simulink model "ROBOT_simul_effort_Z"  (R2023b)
settings: Solver=VariableStepAuto  StartTime=0.0  StopTime=5  RelTol=1e-3
undefined symbols (not defined in the file): deg, kg, m, manette1_Defaut_sldprt, manette2_Defaut_sldprt, mm, N, rad, s, STL, X, Y, Z
libraries: sm_lib x463, fl_lib x45, nesl_utility x27, simulink x2
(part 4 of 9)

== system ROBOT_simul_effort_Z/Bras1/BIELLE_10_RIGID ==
  AXE_BIELLE_1_RIGID : Subsystem
  AXE_BIELLE_2_RIGID : Subsystem
  BIELLE_PARALLELOGRAMME_1_RIGID : Subsystem
  ReferenceFrame : sm_lib/Frames and Transforms/Reference Frame
  Transform : sm_lib/Frames and Transforms/Rigid Transform  TranslationMethod=Cartesian  TranslationStandardOffset=0  TranslationStandardOffsetUnits=mm  TranslationStandardAxis=+Z  TranslationCartesianOffset=[-181.1287710013672 12.999999999999993 -105.75000000000001]  TranslationCartesianOffsetUnits=mm  TranslationROffset=0  TranslationROffsetUnits=m  TranslationZOffset=0  TranslationZOffsetUnits=m  TranslationThetaOffset=0  TranslationThetaOffsetUnits=deg  RotationMethod=ArbitraryAxis  RotationAngleUnits=rad  RotationStandardAxis=+Z  RotationAngle=2.0943951023931957  RotationArbitraryAxis=[0.57735026918962573 -0.57735026918962573 0.57735026918962562]  FollAlignAxisA=+X  BaseAlignAxisA=+Y  FollAlignAxisB=+Y  BaseAlignAxisB=+Z  RotationSequenceAxes=FollowerAxes  RotationSequence=XYX  RotationSequenceAngles=[0 0 0]  RotationSequenceAnglesUnits=deg  RotationMatrix=[1 0 0; 0 1 0; 0 0 1]  Quaternion=[1 0 0 0]
  Transform1 : sm_lib/Frames and Transforms/Rigid Transform  TranslationMethod=Cartesian  TranslationStandardOffset=0  TranslationStandardOffsetUnits=mm  TranslationStandardAxis=+Z  TranslationCartesianOffset=[-181.12877100136717 13.000000000000004 -3.249999999999996]  TranslationCartesianOffsetUnits=mm  TranslationROffset=0  TranslationROffsetUnits=m  TranslationZOffset=0  TranslationZOffsetUnits=m  TranslationThetaOffset=0  TranslationThetaOffsetUnits=deg  RotationMethod=ArbitraryAxis  RotationAngleUnits=rad  RotationStandardAxis=+Z  RotationAngle=2.0943951023931953  RotationArbitraryAxis=[0.57735026918962584 -0.57735026918962584 0.57735026918962584]  FollAlignAxisA=+X  BaseAlignAxisA=+Y  FollAlignAxisB=+Y  BaseAlignAxisB=+Z  RotationSequenceAxes=FollowerAxes  RotationSequence=XYX  RotationSequenceAngles=[0 0 0]  RotationSequenceAnglesUnits=deg  RotationMatrix=[1 0 0; 0 1 0; 0 0 1]  Quaternion=[1 0 0 0]
  Transform2 : sm_lib/Frames and Transforms/Rigid Transform  TranslationMethod=Cartesian  TranslationStandardOffset=0  TranslationStandardOffsetUnits=mm  TranslationStandardAxis=+Z  TranslationCartesianOffset=[-178.12877100136717 5.0000000000000115 -54.500000000000007]  TranslationCartesianOffsetUnits=mm  TranslationROffset=0  TranslationROffsetUnits=m  TranslationZOffset=0  TranslationZOffsetUnits=m  TranslationThetaOffset=0  TranslationThetaOffsetUnits=deg  RotationMethod=ArbitraryAxis  RotationAngleUnits=rad  RotationStandardAxis=+Z  RotationAngle=3.1415926535897931  RotationArbitraryAxis=[-0.70710678118654746 0.70710678118654768 0]  FollAlignAxisA=+X  BaseAlignAxisA=+Y  FollAlignAxisB=+Y  BaseAlignAxisB=+Z  RotationSequenceAxes=FollowerAxes  RotationSequence=XYX  RotationSequenceAngles=[0 0 0]  RotationSequenceAnglesUnits=deg  RotationMatrix=[1 0 0; 0 1 0; 0 0 1]  Quaternion=[1 0 0 0]
  Transform3 : sm_lib/Frames and Transforms/Rigid Transform  TranslationMethod=Cartesian  TranslationStandardOffset=0  TranslationStandardOffsetUnits=mm  TranslationStandardAxis=+Z  TranslationCartesianOffset=[-181.1287710013672 4.999999999999984 -105.75000000000001]  TranslationCartesianOffsetUnits=mm  TranslationROffset=0  TranslationROffsetUnits=m  TranslationZOffset=0  TranslationZOffsetUnits=m  TranslationThetaOffset=0  TranslationThetaOffsetUnits=deg  RotationMethod=ArbitraryAxis  RotationAngleUnits=rad  RotationStandardAxis=+Z  RotationAngle=1.7602050674842988  RotationArbitraryAxis=[-0.82650316451596495 -0.3980530863120495 -0.3980530863120495]  FollAlignAxisA=+X  BaseAlignAxisA=+Y  FollAlignAxisB=+Y  BaseAlignAxisB=+Z  RotationSequenceAxes=FollowerAxes  RotationSequence=XYX  RotationSequenceAngles=[0 0 0]  RotationSequenceAnglesUnits=deg  RotationMatrix=[1 0 0; 0 1 0; 0 0 1]  Quaternion=[1 0 0 0]
  Transform4 : sm_lib/Frames and Transforms/Rigid Transform  TranslationMethod=Cartesian  TranslationStandardOffset=0  TranslationStandardOffsetUnits=mm  TranslationStandardAxis=+Z  TranslationCartesianOffset=[-181.12877100136717 5.0000000000000115 -3.249999999999996]  TranslationCartesianOffsetUnits=mm  TranslationROffset=0  TranslationROffsetUnits=m  TranslationZOffset=0  TranslationZOffsetUnits=m  TranslationThetaOffset=0  TranslationThetaOffsetUnits=deg  RotationMethod=ArbitraryAxis  RotationAngleUnits=rad  RotationStandardAxis=+Z  RotationAngle=1.7602050674842997  RotationArbitraryAxis=[-0.82650316451596506 -0.39805308631204933 -0.39805308631204933]  FollAlignAxisA=+X  BaseAlignAxisA=+Y  FollAlignAxisB=+Y  BaseAlignAxisB=+Z  RotationSequenceAxes=FollowerAxes  RotationSequence=XYX  RotationSequenceAngles=[0 0 0]  RotationSequenceAnglesUnits=deg  RotationMatrix=[1 0 0; 0 1 0; 0 0 1]  Quaternion=[1 0 0 0]
  F1 : PMIOPort  Side=Right
  F : PMIOPort  Port=2  Side=Left
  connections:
  Transform/LConn1 -- ReferenceFrame/RConn1 -- Transform3/LConn1 -- Transform4/LConn1 -- Transform2/LConn1 -- Transform1/LConn1
  Transform/RConn1 -- F/RConn1
  Transform1/RConn1 -- F1/RConn1
  BIELLE_PARALLELOGRAMME_1_RIGID/LConn1 -- Transform2/RConn1
  AXE_BIELLE_1_RIGID/LConn1 -- Transform3/RConn1
  AXE_BIELLE_2_RIGID/LConn1 -- Transform4/RConn1

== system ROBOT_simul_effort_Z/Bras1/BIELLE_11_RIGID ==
  AXE_BIELLE_1_RIGID : Subsystem
  AXE_BIELLE_2_RIGID : Subsystem
  BIELLE_PARALLELOGRAMME_1_RIGID : Subsystem
  ReferenceFrame : sm_lib/Frames and Transforms/Reference Frame
  Transform : sm_lib/Frames and Transforms/Rigid Transform  TranslationMethod=Cartesian  TranslationStandardOffset=0  TranslationStandardOffsetUnits=mm  TranslationStandardAxis=+Z  TranslationCartesianOffset=[-181.12877100136717 13.000000000000018 -105.75000000000001]  TranslationCartesianOffsetUnits=mm  TranslationROffset=0  TranslationROffsetUnits=m  TranslationZOffset=0  TranslationZOffsetUnits=m  TranslationThetaOffset=0  TranslationThetaOffsetUnits=deg  RotationMethod=ArbitraryAxis  RotationAngleUnits=rad  RotationStandardAxis=+Z  RotationAngle=2.0943951023931962  RotationArbitraryAxis=[0.57735026918962595 -0.57735026918962562 0.57735026918962562]  FollAlignAxisA=+X  BaseAlignAxisA=+Y  FollAlignAxisB=+Y  BaseAlignAxisB=+Z  RotationSequenceAxes=FollowerAxes  RotationSequence=XYX  RotationSequenceAngles=[0 0 0]  RotationSequenceAnglesUnits=deg  RotationMatrix=[1 0 0; 0 1 0; 0 0 1]  Quaternion=[1 0 0 0]
  Transform1 : sm_lib/Frames and Transforms/Rigid Transform  TranslationMethod=Cartesian  TranslationStandardOffset=0  TranslationStandardOffsetUnits=mm  TranslationStandardAxis=+Z  TranslationCartesianOffset=[-181.12877100136714 13.000000000000014 -3.2499999999999889]  TranslationCartesianOffsetUnits=mm  TranslationROffset=0  TranslationROffsetUnits=m  TranslationZOffset=0  TranslationZOffsetUnits=m  TranslationThetaOffset=0  TranslationThetaOffsetUnits=deg  RotationMethod=ArbitraryAxis  RotationAngleUnits=rad  RotationStandardAxis=+Z  RotationAngle=2.0943951023931957  RotationArbitraryAxis=[0.57735026918962573 -0.57735026918962562 0.57735026918962595]  FollAlignAxisA=+X  BaseAlignAxisA=+Y  FollAlignAxisB=+Y  BaseAlignAxisB=+Z  RotationSequenceAxes=FollowerAxes  RotationSequence=XYX  RotationSequenceAngles=[0 0 0]  RotationSequenceAnglesUnits=deg  RotationMatrix=[1 0 0; 0 1 0; 0 0 1]  Quaternion=[1 0 0 0]
  Transform2 : sm_lib/Frames and Transforms/Rigid Transform  TranslationMethod=Cartesian  TranslationStandardOffset=0  TranslationStandardOffsetUnits=mm  TranslationStandardAxis=+Z  TranslationCartesianOffset=[-178.12877100136714 5.0000000000000044 -54.500000000000007]  TranslationCartesianOffsetUnits=mm  TranslationROffset=0  TranslationROffsetUnits=m  TranslationZOffset=0  TranslationZOffsetUnits=m  TranslationThetaOffset=0  TranslationThetaOffsetUnits=deg  RotationMethod=ArbitraryAxis  RotationAngleUnits=rad  RotationStandardAxis=+Z  RotationAngle=3.1415926535897931  RotationArbitraryAxis=[-0.70710678118654746 0.70710678118654757 0]  FollAlignAxisA=+X  BaseAlignAxisA=+Y  FollAlignAxisB=+Y  BaseAlignAxisB=+Z  RotationSequenceAxes=FollowerAxes  RotationSequence=XYX  RotationSequenceAngles=[0 0 0]  RotationSequenceAnglesUnits=deg  RotationMatrix=[1 0 0; 0 1 0; 0 0 1]  Quaternion=[1 0 0 0]
  Transform3 : sm_lib/Frames and Transforms/Rigid Transform  TranslationMethod=Cartesian  TranslationStandardOffset=0  TranslationStandardOffsetUnits=mm  TranslationStandardAxis=+Z  TranslationCartesianOffset=[-181.12877100136717 5.0000000000000044 -105.75000000000001]  TranslationCartesianOffsetUnits=mm  TranslationROffset=0  TranslationROffsetUnits=m  TranslationZOffset=0  TranslationZOffsetUnits=m  TranslationThetaOffset=0  TranslationThetaOffsetUnits=deg  RotationMethod=ArbitraryAxis  RotationAngleUnits=rad  RotationStandardAxis=+Z  RotationAngle=1.7602050674842991  RotationArbitraryAxis=[-0.82650316451596495 -0.3980530863120495 -0.39805308631204944]  FollAlignAxisA=+X  BaseAlignAxisA=+Y  FollAlignAxisB=+Y  BaseAlignAxisB=+Z  RotationSequenceAxes=FollowerAxes  RotationSequence=XYX  RotationSequenceAngles=[0 0 0]  RotationSequenceAnglesUnits=deg  RotationMatrix=[1 0 0; 0 1 0; 0 0 1]  Quaternion=[1 0 0 0]
  Transform4 : sm_lib/Frames and Transforms/Rigid Transform  TranslationMethod=Cartesian  TranslationStandardOffset=0  TranslationStandardOffsetUnits=mm  TranslationStandardAxis=+Z  TranslationCartesianOffset=[-181.12877100136714 5.0000000000000044 -3.2499999999999889]  TranslationCartesianOffsetUnits=mm  TranslationROffset=0  TranslationROffsetUnits=m  TranslationZOffset=0  TranslationZOffsetUnits=m  TranslationThetaOffset=0  TranslationThetaOffsetUnits=deg  RotationMethod=ArbitraryAxis  RotationAngleUnits=rad  RotationStandardAxis=+Z  RotationAngle=1.7602050674842995  RotationArbitraryAxis=[-0.82650316451596506 -0.39805308631204939 -0.39805308631204933]  FollAlignAxisA=+X  BaseAlignAxisA=+Y  FollAlignAxisB=+Y  BaseAlignAxisB=+Z  RotationSequenceAxes=FollowerAxes  RotationSequence=XYX  RotationSequenceAngles=[0 0 0]  RotationSequenceAnglesUnits=deg  RotationMatrix=[1 0 0; 0 1 0; 0 0 1]  Quaternion=[1 0 0 0]
  F1 : PMIOPort  Side=Right
  F : PMIOPort  Port=2  Side=Left
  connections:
  Transform/LConn1 -- ReferenceFrame/RConn1 -- Transform3/LConn1 -- Transform4/LConn1 -- Transform2/LConn1 -- Transform1/LConn1
  Transform/RConn1 -- F/RConn1
  Transform1/RConn1 -- F1/RConn1
  BIELLE_PARALLELOGRAMME_1_RIGID/LConn1 -- Transform2/RConn1
  AXE_BIELLE_1_RIGID/LConn1 -- Transform3/RConn1
  AXE_BIELLE_2_RIGID/LConn1 -- Transform4/RConn1

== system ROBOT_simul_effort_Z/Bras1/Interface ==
  Angular Velocity Source : fl_lib/Mechanical/Mechanical Sources/Ideal Angular Velocity Source
  Torque Sensor : fl_lib/Mechanical/Mechanical Sensors/Ideal Torque Sensor
  C : PMIOPort  Side=Left
  T : PMIOPort  Port=2  Side=Right
  w : PMIOPort  Port=3  Side=Right
  R : PMIOPort  Port=4  Side=Left
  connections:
  R/RConn1 -- Angular Velocity Source/LConn1
  Torque Sensor/LConn1 -- Angular Velocity Source/RConn2
  Torque Sensor/RConn2 -- T/RConn1
  C/RConn1 -- Torque Sensor/RConn1
  Angular Velocity Source/RConn1 -- w/RConn1

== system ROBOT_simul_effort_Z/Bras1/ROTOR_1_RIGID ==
  CODEUR_1_RIGID : Subsystem
  ROTOR_1_RIGID : Subsystem
  ReferenceFrame : sm_lib/Frames and Transforms/Reference Frame
  Transform : sm_lib/Frames and Transforms/Rigid Transform  TranslationMethod=Cartesian  TranslationStandardOffset=0  TranslationStandardOffsetUnits=mm  TranslationStandardAxis=+Z  TranslationCartesianOffset=[29.900000000000013 -3.5527136788005009e-15 2.2204460492503131e-14]  TranslationCartesianOffsetUnits=mm  TranslationROffset=0  TranslationROffsetUnits=m  TranslationZOffset=0  TranslationZOffsetUnits=m  TranslationThetaOffset=0  TranslationThetaOffsetUnits=deg  RotationMethod=ArbitraryAxis  RotationAngleUnits=rad  RotationStandardAxis=+Z  RotationAngle=2.0943951023931953  RotationArbitraryAxis=[0.57735026918962595 0.57735026918962562 0.57735026918962562]  FollAlignAxisA=+X  BaseAlignAxisA=+Y  FollAlignAxisB=+Y  BaseAlignAxisB=+Z  RotationSequenceAxes=FollowerAxes  RotationSequence=XYX  RotationSequenceAngles=[0 0 0]  RotationSequenceAnglesUnits=deg  RotationMatrix=[1 0 0; 0 1 0; 0 0 1]  Quaternion=[1 0 0 0]
  Transform1 : sm_lib/Frames and Transforms/Rigid Transform  TranslationMethod=Cartesian  TranslationStandardOffset=0  TranslationStandardOffsetUnits=mm  TranslationStandardAxis=+Z  TranslationCartesianOffset=[30.899999999999981 0 0]  TranslationCartesianOffsetUnits=mm  TranslationROffset=0  TranslationROffsetUnits=m  TranslationZOffset=0  TranslationZOffsetUnits=m  TranslationThetaOffset=0  TranslationThetaOffsetUnits=deg  RotationMethod=ArbitraryAxis  RotationAngleUnits=rad  RotationStandardAxis=+Z  RotationAngle=1.9381695666920586  RotationArbitraryAxis=[0.51405666735189148 -0.51405666735189148 0.68665237602598705]  FollAlignAxisA=+X  BaseAlignAxisA=+Y  FollAlignAxisB=+Y  BaseAlignAxisB=+Z  RotationSequenceAxes=FollowerAxes  RotationSequence=XYX  RotationSequenceAngles=[0 0 0]  RotationSequenceAnglesUnits=deg  RotationMatrix=[1 0 0; 0 1 0; 0 0 1]  Quaternion=[1 0 0 0]
  Transform2 : sm_lib/Frames and Transforms/Rigid Transform  TranslationMethod=Cartesian  TranslationStandardOffset=0  TranslationStandardOffsetUnits=mm  TranslationStandardAxis=+Z  TranslationCartesianOffset=[-36.399999999999999 0 0]  TranslationCartesianOffsetUnits=mm  TranslationROffset=0  TranslationROffsetUnits=m  TranslationZOffset=0  TranslationZOffsetUnits=m  TranslationThetaOffset=0  TranslationThetaOffsetUnits=deg  RotationMethod=ArbitraryAxis  RotationAngleUnits=rad  RotationStandardAxis=+Z  RotationAngle=1.624664356272121  RotationArbitraryAxis=[-0.22603347840136145 0.22603347840136123 0.94753244444903439]  FollAlignAxisA=+X  BaseAlignAxisA=+Y  FollAlignAxisB=+Y  BaseAlignAxisB=+Z  RotationSequenceAxes=FollowerAxes  RotationSequence=XYX  RotationSequenceAngles=[0 0 0]  RotationSequenceAnglesUnits=deg  RotationMatrix=[1 0 0; 0 1 0; 0 0 1]  Quaternion=[1 0 0 0]
  F : PMIOPort  Side=Left
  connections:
  Transform/LConn1 -- ReferenceFrame/RConn1 -- Transform1/LConn1 -- Transform2/LConn1
  Transform/RConn1 -- F/RConn1
  ROTOR_1_RIGID/LConn1 -- Transform1/RConn1
  CODEUR_1_RIGID/LConn1 -- Transform2/RConn1

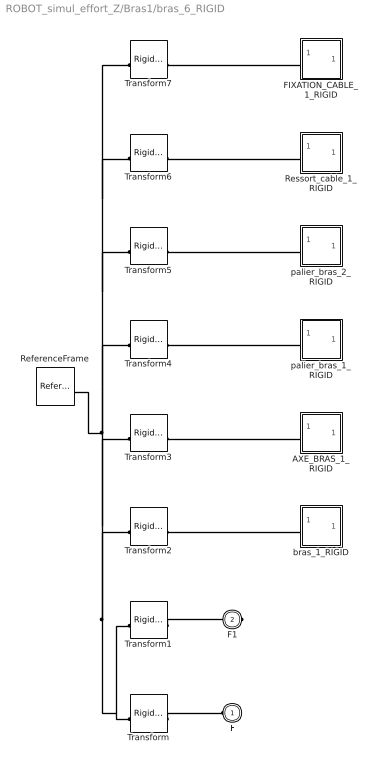
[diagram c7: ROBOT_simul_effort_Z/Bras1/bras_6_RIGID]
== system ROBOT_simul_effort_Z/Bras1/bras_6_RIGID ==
  AXE_BRAS_1_RIGID : Subsystem
  FIXATION_CABLE_1_RIGID : Subsystem
  ReferenceFrame : sm_lib/Frames and Transforms/Reference Frame
  Ressort_cable_1_RIGID : Subsystem
  Transform : sm_lib/Frames and Transforms/Rigid Transform  TranslationMethod=Cartesian  TranslationStandardOffset=0  TranslationStandardOffsetUnits=mm  TranslationStandardAxis=+Z  TranslationCartesianOffset=[-97.415569487383038 39.82561820207529 -20.980989744699272]  TranslationCartesianOffsetUnits=mm  TranslationROffset=0  TranslationROffsetUnits=m  TranslationZOffset=0  TranslationZOffsetUnits=m  TranslationThetaOffset=0  TranslationThetaOffsetUnits=deg  RotationMethod=ArbitraryAxis  RotationAngleUnits=rad  RotationStandardAxis=+Z  RotationAngle=2.0943951023931957  RotationArbitraryAxis=[-0.57735026918962551 -0.57735026918962595 0.57735026918962573]  FollAlignAxisA=+X  BaseAlignAxisA=+Y  FollAlignAxisB=+Y  BaseAlignAxisB=+Z  RotationSequenceAxes=FollowerAxes  RotationSequence=XYX  RotationSequenceAngles=[0 0 0]  RotationSequenceAnglesUnits=deg  RotationMatrix=[1 0 0; 0 1 0; 0 0 1]  Quaternion=[1 0 0 0]
  Transform1 : sm_lib/Frames and Transforms/Rigid Transform  TranslationMethod=Cartesian  TranslationStandardOffset=0  TranslationStandardOffsetUnits=mm  TranslationStandardAxis=+Z  TranslationCartesianOffset=[-176.59192436800635 99.825618202078147 -20.980989744703663]  TranslationCartesianOffsetUnits=mm  TranslationROffset=0  TranslationROffsetUnits=m  TranslationZOffset=0  TranslationZOffsetUnits=m  TranslationThetaOffset=0  TranslationThetaOffsetUnits=deg  RotationMethod=ArbitraryAxis  RotationAngleUnits=rad  RotationStandardAxis=+Z  RotationAngle=2.0943951023931953  RotationArbitraryAxis=[0.57735026918962584 0.57735026918962584 0.57735026918962584]  FollAlignAxisA=+X  BaseAlignAxisA=+Y  FollAlignAxisB=+Y  BaseAlignAxisB=+Z  RotationSequenceAxes=FollowerAxes  RotationSequence=XYX  RotationSequenceAngles=[0 0 0]  RotationSequenceAnglesUnits=deg  RotationMatrix=[1 0 0; 0 1 0; 0 0 1]  Quaternion=[1 0 0 0]
  Transform2 : sm_lib/Frames and Transforms/Rigid Transform  TranslationMethod=Cartesian  TranslationStandardOffset=0  TranslationStandardOffsetUnits=mm  TranslationStandardAxis=+Z  TranslationCartesianOffset=[-166.59192436800635 39.825618202078147 -20.98098974470366]  TranslationCartesianOffsetUnits=mm  TranslationROffset=0  TranslationROffsetUnits=m  TranslationZOffset=0  TranslationZOffsetUnits=m  TranslationThetaOffset=0  TranslationThetaOffsetUnits=deg  RotationMethod=ArbitraryAxis  RotationAngleUnits=rad  RotationStandardAxis=+Z  RotationAngle=1.5707963267948968  RotationArbitraryAxis=[-0 -1 -0]  FollAlignAxisA=+X  BaseAlignAxisA=+Y  FollAlignAxisB=+Y  BaseAlignAxisB=+Z  RotationSequenceAxes=FollowerAxes  RotationSequence=XYX  RotationSequenceAngles=[0 0 0]  RotationSequenceAnglesUnits=deg  RotationMatrix=[1 0 0; 0 1 0; 0 0 1]  Quaternion=[1 0 0 0]
  Transform3 : sm_lib/Frames and Transforms/Rigid Transform  TranslationMethod=Cartesian  TranslationStandardOffset=0  TranslationStandardOffsetUnits=mm  TranslationStandardAxis=+Z  TranslationCartesianOffset=[-166.59192436800635 39.825618202078147 -20.98098974470366]  TranslationCartesianOffsetUnits=mm  TranslationROffset=0  TranslationROffsetUnits=m  TranslationZOffset=0  TranslationZOffsetUnits=m  TranslationThetaOffset=0  TranslationThetaOffsetUnits=deg  RotationMethod=ArbitraryAxis  RotationAngleUnits=rad  RotationStandardAxis=+Z  RotationAngle=1.5707963267948968  RotationArbitraryAxis=[0 1 0]  FollAlignAxisA=+X  BaseAlignAxisA=+Y  FollAlignAxisB=+Y  BaseAlignAxisB=+Z  RotationSequenceAxes=FollowerAxes  RotationSequence=XYX  RotationSequenceAngles=[0 0 0]  RotationSequenceAnglesUnits=deg  RotationMatrix=[1 0 0; 0 1 0; 0 0 1]  Quaternion=[1 0 0 0]
  Transform4 : sm_lib/Frames and Transforms/Rigid Transform  TranslationMethod=None  TranslationStandardOffset=0  TranslationStandardOffsetUnits=m  TranslationStandardAxis=+Z  TranslationCartesianOffset=[0 0 0]  TranslationCartesianOffsetUnits=m  TranslationROffset=0  TranslationROffsetUnits=m  TranslationZOffset=0  TranslationZOffsetUnits=m  TranslationThetaOffset=0  TranslationThetaOffsetUnits=deg  RotationMethod=None  RotationAngleUnits=deg  RotationStandardAxis=+Z  RotationAngle=0  RotationArbitraryAxis=[0 0 1]  FollAlignAxisA=+X  BaseAlignAxisA=+Y  FollAlignAxisB=+Y  BaseAlignAxisB=+Z  RotationSequenceAxes=FollowerAxes  RotationSequence=XYX  RotationSequenceAngles=[0 0 0]  RotationSequenceAnglesUnits=deg  RotationMatrix=[1 0 0; 0 1 0; 0 0 1]  Quaternion=[1 0 0 0]
  Transform5 : sm_lib/Frames and Transforms/Rigid Transform  TranslationMethod=Cartesian  TranslationStandardOffset=0  TranslationStandardOffsetUnits=mm  TranslationStandardAxis=+Z  TranslationCartesianOffset=[-333.18384873601275 5.2270863233389582 7.8152493791980238]  TranslationCartesianOffsetUnits=mm  TranslationROffset=0  TranslationROffsetUnits=m  TranslationZOffset=0  TranslationZOffsetUnits=m  TranslationThetaOffset=0  TranslationThetaOffsetUnits=deg  RotationMethod=ArbitraryAxis  RotationAngleUnits=rad  RotationStandardAxis=+Z  RotationAngle=3.1415926535897931  RotationArbitraryAxis=[0 0.83121877946981937 -0.55594544755461728]  FollAlignAxisA=+X  BaseAlignAxisA=+Y  FollAlignAxisB=+Y  BaseAlignAxisB=+Z  RotationSequenceAxes=FollowerAxes  RotationSequence=XYX  RotationSequenceAngles=[0 0 0]  RotationSequenceAnglesUnits=deg  RotationMatrix=[1 0 0; 0 1 0; 0 0 1]  Quaternion=[1 0 0 0]
  Transform6 : sm_lib/Frames and Transforms/Rigid Transform  TranslationMethod=Cartesian  TranslationStandardOffset=0  TranslationStandardOffsetUnits=mm  TranslationStandardAxis=+Z  TranslationCartesianOffset=[-166.59192436800637 17.182941135267072 -24.980989744703663]  TranslationCartesianOffsetUnits=mm  TranslationROffset=0  TranslationROffsetUnits=m  TranslationZOffset=0  TranslationZOffsetUnits=m  TranslationThetaOffset=0  TranslationThetaOffsetUnits=deg  RotationMethod=ArbitraryAxis  RotationAngleUnits=rad  RotationStandardAxis=+Z  RotationAngle=1.5707963267948968  RotationArbitraryAxis=[1 0 0]  FollAlignAxisA=+X  BaseAlignAxisA=+Y  FollAlignAxisB=+Y  BaseAlignAxisB=+Z  RotationSequenceAxes=FollowerAxes  RotationSequence=XYX  RotationSequenceAngles=[0 0 0]  RotationSequenceAnglesUnits=deg  RotationMatrix=[1 0 0; 0 1 0; 0 0 1]  Quaternion=[1 0 0 0]
  Transform7 : sm_lib/Frames and Transforms/Rigid Transform  TranslationMethod=Cartesian  TranslationStandardOffset=0  TranslationStandardOffsetUnits=mm  TranslationStandardAxis=+Z  TranslationCartesianOffset=[-172.59192436800637 90.586314327933906 3.4188407632840327]  TranslationCartesianOffsetUnits=mm  TranslationROffset=0  TranslationROffsetUnits=m  TranslationZOffset=0  TranslationZOffsetUnits=m  TranslationThetaOffset=0  TranslationThetaOffsetUnits=deg  RotationMethod=ArbitraryAxis  RotationAngleUnits=rad  RotationStandardAxis=+Z  RotationAngle=1.0159852938148253  RotationArbitraryAxis=[-1 0 0]  FollAlignAxisA=+X  BaseAlignAxisA=+Y  FollAlignAxisB=+Y  BaseAlignAxisB=+Z  RotationSequenceAxes=FollowerAxes  RotationSequence=XYX  RotationSequenceAngles=[0 0 0]  RotationSequenceAnglesUnits=deg  RotationMatrix=[1 0 0; 0 1 0; 0 0 1]  Quaternion=[1 0 0 0]
  bras_1_RIGID : Subsystem
  palier_bras_1_RIGID : Subsystem
  palier_bras_2_RIGID : Subsystem
  F : PMIOPort  Side=Left
  F1 : PMIOPort  Port=2  Side=Right
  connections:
  Transform/LConn1 -- ReferenceFrame/RConn1 -- Transform6/LConn1 -- Transform7/LConn1 -- Transform5/LConn1 -- Transform4/LConn1 -- Transform3/LConn1 -- Transform2/LConn1 -- Transform1/LConn1
  Transform/RConn1 -- F/RConn1
  Transform1/RConn1 -- F1/RConn1
  Transform2/RConn1 -- bras_1_RIGID/LConn1
  AXE_BRAS_1_RIGID/LConn1 -- Transform3/RConn1
  Transform4/RConn1 -- palier_bras_1_RIGID/LConn1
  Transform5/RConn1 -- palier_bras_2_RIGID/LConn1
  Ressort_cable_1_RIGID/LConn1 -- Transform6/RConn1
  FIXATION_CABLE_1_RIGID/LConn1 -- Transform7/RConn1

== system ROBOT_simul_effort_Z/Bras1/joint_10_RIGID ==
  AXE_BRAS_1_RIGID : Subsystem
  ReferenceFrame : sm_lib/Frames and Transforms/Reference Frame
  Transform : sm_lib/Frames and Transforms/Rigid Transform  TranslationMethod=Cartesian  TranslationStandardOffset=0  TranslationStandardOffsetUnits=mm  TranslationStandardAxis=+Z  TranslationCartesianOffset=[-153.62772197331242 116.19029839316632 -133.8263224253264]  TranslationCartesianOffsetUnits=mm  TranslationROffset=0  TranslationROffsetUnits=m  TranslationZOffset=0  TranslationZOffsetUnits=m  TranslationThetaOffset=0  TranslationThetaOffsetUnits=deg  RotationMethod=ArbitraryAxis  RotationAngleUnits=rad  RotationStandardAxis=+Z  RotationAngle=1.9754511492118261  RotationArbitraryAxis=[-0.53149434051907762 -0.53149434051907807 -0.65956616953295977]  FollAlignAxisA=+X  BaseAlignAxisA=+Y  FollAlignAxisB=+Y  BaseAlignAxisB=+Z  RotationSequenceAxes=FollowerAxes  RotationSequence=XYX  RotationSequenceAngles=[0 0 0]  RotationSequenceAnglesUnits=deg  RotationMatrix=[1 0 0; 0 1 0; 0 0 1]  Quaternion=[1 0 0 0]
  Transform1 : sm_lib/Frames and Transforms/Rigid Transform  TranslationMethod=Cartesian  TranslationStandardOffset=0  TranslationStandardOffsetUnits=mm  TranslationStandardAxis=+Z  TranslationCartesianOffset=[-181.62772197331248 131.82453775326121 -130.42476989284125]  TranslationCartesianOffsetUnits=mm  TranslationROffset=0  TranslationROffsetUnits=m  TranslationZOffset=0  TranslationZOffsetUnits=m  TranslationThetaOffset=0  TranslationThetaOffsetUnits=deg  RotationMethod=ArbitraryAxis  RotationAngleUnits=rad  RotationStandardAxis=+Z  RotationAngle=2.2221940470110657  RotationArbitraryAxis=[0.61437017396793003 -0.61437017396792981 0.49507431631749077]  FollAlignAxisA=+X  BaseAlignAxisA=+Y  FollAlignAxisB=+Y  BaseAlignAxisB=+Z  RotationSequenceAxes=FollowerAxes  RotationSequence=XYX  RotationSequenceAngles=[0 0 0]  RotationSequenceAnglesUnits=deg  RotationMatrix=[1 0 0; 0 1 0; 0 0 1]  Quaternion=[1 0 0 0]
  Transform2 : sm_lib/Frames and Transforms/Rigid Transform  TranslationMethod=Cartesian  TranslationStandardOffset=0  TranslationStandardOffsetUnits=mm  TranslationStandardAxis=+Z  TranslationCartesianOffset=[-177.62772197331233 126.39913469761095 -143.1183707091472]  TranslationCartesianOffsetUnits=mm  TranslationROffset=0  TranslationROffsetUnits=m  TranslationZOffset=0  TranslationZOffsetUnits=m  TranslationThetaOffset=0  TranslationThetaOffsetUnits=deg  RotationMethod=ArbitraryAxis  RotationAngleUnits=rad  RotationStandardAxis=+Z  RotationAngle=2.0943951023931957  RotationArbitraryAxis=[0.57735026918962551 0.57735026918962584 0.57735026918962595]  FollAlignAxisA=+X  BaseAlignAxisA=+Y  FollAlignAxisB=+Y  BaseAlignAxisB=+Z  RotationSequenceAxes=FollowerAxes  RotationSequence=XYX  RotationSequenceAngles=[0 0 0]  RotationSequenceAnglesUnits=deg  RotationMatrix=[1 0 0; 0 1 0; 0 0 1]  Quaternion=[1 0 0 0]
  Transform3 : sm_lib/Frames and Transforms/Rigid Transform  TranslationMethod=Cartesian  TranslationStandardOffset=0  TranslationStandardOffsetUnits=mm  TranslationStandardAxis=+Z  TranslationCartesianOffset=[-167.62772197331245 128.09991096385986 -150.93549038919826]  TranslationCartesianOffsetUnits=mm  TranslationROffset=0  TranslationROffsetUnits=m  TranslationZOffset=0  TranslationZOffsetUnits=m  TranslationThetaOffset=0  TranslationThetaOffsetUnits=deg  RotationMethod=ArbitraryAxis  RotationAngleUnits=rad  RotationStandardAxis=+Z  RotationAngle=1.7850283121554718  RotationArbitraryAxis=[1 7.8579866763579256e-16 -6.7960803884612889e-16]  FollAlignAxisA=+X  BaseAlignAxisA=+Y  FollAlignAxisB=+Y  BaseAlignAxisB=+Z  RotationSequenceAxes=FollowerAxes  RotationSequence=XYX  RotationSequenceAngles=[0 0 0]  RotationSequenceAnglesUnits=deg  RotationMatrix=[1 0 0; 0 1 0; 0 0 1]  Quaternion=[1 0 0 0]
  Transform4 : sm_lib/Frames and Transforms/Rigid Transform  TranslationMethod=Cartesian  TranslationStandardOffset=0  TranslationStandardOffsetUnits=mm  TranslationStandardAxis=+Z  TranslationCartesianOffset=[-167.62772197331239 126.39913469761737 -143.11837070915072]  TranslationCartesianOffsetUnits=mm  TranslationROffset=0  TranslationROffsetUnits=m  TranslationZOffset=0  TranslationZOffsetUnits=m  TranslationThetaOffset=0  TranslationThetaOffsetUnits=deg  RotationMethod=ArbitraryAxis  RotationAngleUnits=rad  RotationStandardAxis=+Z  RotationAngle=1.5707963267948968  RotationArbitraryAxis=[-0 -1 -0]  FollAlignAxisA=+X  BaseAlignAxisA=+Y  FollAlignAxisB=+Y  BaseAlignAxisB=+Z  RotationSequenceAxes=FollowerAxes  RotationSequence=XYX  RotationSequenceAngles=[0 0 0]  RotationSequenceAnglesUnits=deg  RotationMatrix=[1 0 0; 0 1 0; 0 0 1]  Quaternion=[1 0 0 0]
  joint_1_RIGID : Subsystem
  F2 : PMIOPort  Side=Left
  F1 : PMIOPort  Port=2  Side=Right
  F : PMIOPort  Port=3  Side=Right
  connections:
  Transform/LConn1 -- ReferenceFrame/RConn1 -- Transform3/LConn1 -- Transform4/LConn1 -- Transform2/LConn1 -- Transform1/LConn1
  Transform/RConn1 -- F/RConn1
  Transform1/RConn1 -- F1/RConn1
  Transform2/RConn1 -- F2/RConn1
  Transform3/RConn1 -- joint_1_RIGID/LConn1
  AXE_BRAS_1_RIGID/LConn1 -- Transform4/RConn1

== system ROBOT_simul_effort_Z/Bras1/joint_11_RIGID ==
  AXE_BRAS_1_RIGID : Subsystem
  ReferenceFrame : sm_lib/Frames and Transforms/Reference Frame
  Transform : sm_lib/Frames and Transforms/Rigid Transform  TranslationMethod=Cartesian  TranslationStandardOffset=0  TranslationStandardOffsetUnits=mm  TranslationStandardAxis=+Z  TranslationCartesianOffset=[-153.62772197331219 131.82453775326144 -130.42476989284148]  TranslationCartesianOffsetUnits=mm  TranslationROffset=0  TranslationROffsetUnits=m  TranslationZOffset=0  TranslationZOffsetUnits=m  TranslationThetaOffset=0  TranslationThetaOffsetUnits=deg  RotationMethod=ArbitraryAxis  RotationAngleUnits=rad  RotationStandardAxis=+Z  RotationAngle=2.2221940470110675  RotationArbitraryAxis=[0.61437017396793037 -0.61437017396793037 0.49507431631748977]  FollAlignAxisA=+X  BaseAlignAxisA=+Y  FollAlignAxisB=+Y  BaseAlignAxisB=+Z  RotationSequenceAxes=FollowerAxes  RotationSequence=XYX  RotationSequenceAngles=[0 0 0]  RotationSequenceAnglesUnits=deg  RotationMatrix=[1 0 0; 0 1 0; 0 0 1]  Quaternion=[1 0 0 0]
  Transform1 : sm_lib/Frames and Transforms/Rigid Transform  TranslationMethod=Cartesian  TranslationStandardOffset=0  TranslationStandardOffsetUnits=mm  TranslationStandardAxis=+Z  TranslationCartesianOffset=[-181.62772197331228 116.19029839316632 -133.82632242532665]  TranslationCartesianOffsetUnits=mm  TranslationROffset=0  TranslationROffsetUnits=m  TranslationZOffset=0  TranslationZOffsetUnits=m  TranslationThetaOffset=0  TranslationThetaOffsetUnits=deg  RotationMethod=ArbitraryAxis  RotationAngleUnits=rad  RotationStandardAxis=+Z  RotationAngle=1.9754511492118272  RotationArbitraryAxis=[-0.53149434051907796 -0.53149434051907796 -0.65956616953295966]  FollAlignAxisA=+X  BaseAlignAxisA=+Y  FollAlignAxisB=+Y  BaseAlignAxisB=+Z  RotationSequenceAxes=FollowerAxes  RotationSequence=XYX  RotationSequenceAngles=[0 0 0]  RotationSequenceAnglesUnits=deg  RotationMatrix=[1 0 0; 0 1 0; 0 0 1]  Quaternion=[1 0 0 0]
  Transform2 : sm_lib/Frames and Transforms/Rigid Transform  TranslationMethod=Cartesian  TranslationStandardOffset=0  TranslationStandardOffsetUnits=mm  TranslationStandardAxis=+Z  TranslationCartesianOffset=[-186.51855936809574 126.39913469761754 -143.11837070915104]  TranslationCartesianOffsetUnits=mm  TranslationROffset=0  TranslationROffsetUnits=m  TranslationZOffset=0  TranslationZOffsetUnits=m  TranslationThetaOffset=0  TranslationThetaOffsetUnits=deg  RotationMethod=ArbitraryAxis  RotationAngleUnits=rad  RotationStandardAxis=+Z  RotationAngle=2.0943951023931904  RotationArbitraryAxis=[0.57735026918962595 0.57735026918962407 0.57735026918962729]  FollAlignAxisA=+X  BaseAlignAxisA=+Y  FollAlignAxisB=+Y  BaseAlignAxisB=+Z  RotationSequenceAxes=FollowerAxes  RotationSequence=XYX  RotationSequenceAngles=[0 0 0]  RotationSequenceAnglesUnits=deg  RotationMatrix=[1 0 0; 0 1 0; 0 0 1]  Quaternion=[1 0 0 0]
  Transform3 : sm_lib/Frames and Transforms/Rigid Transform  TranslationMethod=Cartesian  TranslationStandardOffset=0  TranslationStandardOffsetUnits=mm  TranslationStandardAxis=+Z  TranslationCartesianOffset=[-167.62772197331245 128.09991096385986 -150.93549038919824]  TranslationCartesianOffsetUnits=mm  TranslationROffset=0  TranslationROffsetUnits=m  TranslationZOffset=0  TranslationZOffsetUnits=m  TranslationThetaOffset=0  TranslationThetaOffsetUnits=deg  RotationMethod=ArbitraryAxis  RotationAngleUnits=rad  RotationStandardAxis=+Z  RotationAngle=1.7850283121554718  RotationArbitraryAxis=[1 8.1463180608813852e-16 -6.9713561493488163e-16]  FollAlignAxisA=+X  BaseAlignAxisA=+Y  FollAlignAxisB=+Y  BaseAlignAxisB=+Z  RotationSequenceAxes=FollowerAxes  RotationSequence=XYX  RotationSequenceAngles=[0 0 0]  RotationSequenceAnglesUnits=deg  RotationMatrix=[1 0 0; 0 1 0; 0 0 1]  Quaternion=[1 0 0 0]
  Transform4 : sm_lib/Frames and Transforms/Rigid Transform  TranslationMethod=Cartesian  TranslationStandardOffset=0  TranslationStandardOffsetUnits=mm  TranslationStandardAxis=+Z  TranslationCartesianOffset=[-167.62772197331239 126.39913469761737 -143.11837070915067]  TranslationCartesianOffsetUnits=mm  TranslationROffset=0  TranslationROffsetUnits=m  TranslationZOffset=0  TranslationZOffsetUnits=m  TranslationThetaOffset=0  TranslationThetaOffsetUnits=deg  RotationMethod=ArbitraryAxis  RotationAngleUnits=rad  RotationStandardAxis=+Z  RotationAngle=1.5707963267948968  RotationArbitraryAxis=[-5.5511151231257821e-17 -1 -5.5511151231257821e-17]  FollAlignAxisA=+X  BaseAlignAxisA=+Y  FollAlignAxisB=+Y  BaseAlignAxisB=+Z  RotationSequenceAxes=FollowerAxes  RotationSequence=XYX  RotationSequenceAngles=[0 0 0]  RotationSequenceAnglesUnits=deg  RotationMatrix=[1 0 0; 0 1 0; 0 0 1]  Quaternion=[1 0 0 0]
  joint_1_RIGID : Subsystem
  F2 : PMIOPort  Side=Right
  F1 : PMIOPort  Port=2  Side=Left
  F : PMIOPort  Port=3  Side=Left
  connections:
  Transform/LConn1 -- ReferenceFrame/RConn1 -- Transform3/LConn1 -- Transform4/LConn1 -- Transform2/LConn1 -- Transform1/LConn1
  Transform/RConn1 -- F/RConn1
  Transform1/RConn1 -- F1/RConn1
  Transform2/RConn1 -- F2/RConn1
  Transform3/RConn1 -- joint_1_RIGID/LConn1
  AXE_BRAS_1_RIGID/LConn1 -- Transform4/RConn1

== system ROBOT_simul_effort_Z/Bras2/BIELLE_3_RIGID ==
  AXE_BIELLE_1_RIGID : Subsystem
  AXE_BIELLE_2_RIGID : Subsystem
  BIELLE_PARALLELOGRAMME_1_RIGID : Subsystem
  ReferenceFrame : sm_lib/Frames and Transforms/Reference Frame
  Transform : sm_lib/Frames and Transforms/Rigid Transform  TranslationMethod=Cartesian  TranslationStandardOffset=0  TranslationStandardOffsetUnits=mm  TranslationStandardAxis=+Z  TranslationCartesianOffset=[-181.12877100137212 -3.0000000000000853 -105.74999999999531]  TranslationCartesianOffsetUnits=mm  TranslationROffset=0  TranslationROffsetUnits=m  TranslationZOffset=0  TranslationZOffsetUnits=m  TranslationThetaOffset=0  TranslationThetaOffsetUnits=deg  RotationMethod=ArbitraryAxis  RotationAngleUnits=rad  RotationStandardAxis=+Z  RotationAngle=2.0943951023931957  RotationArbitraryAxis=[-0.57735026918962584 -0.57735026918962573 -0.57735026918962573]  FollAlignAxisA=+X  BaseAlignAxisA=+Y  FollAlignAxisB=+Y  BaseAlignAxisB=+Z  RotationSequenceAxes=FollowerAxes  RotationSequence=XYX  RotationSequenceAngles=[0 0 0]  RotationSequenceAnglesUnits=deg  RotationMatrix=[1 0 0; 0 1 0; 0 0 1]  Quaternion=[1 0 0 0]
  Transform1 : sm_lib/Frames and Transforms/Rigid Transform  TranslationMethod=Cartesian  TranslationStandardOffset=0  TranslationStandardOffsetUnits=mm  TranslationStandardAxis=+Z  TranslationCartesianOffset=[-181.12877100136708 12.999999999999984 -3.2500000000000027]  TranslationCartesianOffsetUnits=mm  TranslationROffset=0  TranslationROffsetUnits=m  TranslationZOffset=0  TranslationZOffsetUnits=m  TranslationThetaOffset=0  TranslationThetaOffsetUnits=deg  RotationMethod=ArbitraryAxis  RotationAngleUnits=rad  RotationStandardAxis=+Z  RotationAngle=2.0943951023931953  RotationArbitraryAxis=[0.57735026918962584 -0.57735026918962584 0.57735026918962584]  FollAlignAxisA=+X  BaseAlignAxisA=+Y  FollAlignAxisB=+Y  BaseAlignAxisB=+Z  RotationSequenceAxes=FollowerAxes  RotationSequence=XYX  RotationSequenceAngles=[0 0 0]  RotationSequenceAnglesUnits=deg  RotationMatrix=[1 0 0; 0 1 0; 0 0 1]  Quaternion=[1 0 0 0]
  Transform2 : sm_lib/Frames and Transforms/Rigid Transform  TranslationMethod=Cartesian  TranslationStandardOffset=0  TranslationStandardOffsetUnits=mm  TranslationStandardAxis=+Z  TranslationCartesianOffset=[-178.12877100136706 4.9999999999999902 -54.499999999999957]  TranslationCartesianOffsetUnits=mm  TranslationROffset=0  TranslationROffsetUnits=m  TranslationZOffset=0  TranslationZOffsetUnits=m  TranslationThetaOffset=0  TranslationThetaOffsetUnits=deg  RotationMethod=ArbitraryAxis  RotationAngleUnits=rad  RotationStandardAxis=+Z  RotationAngle=3.1415926535897931  RotationArbitraryAxis=[-0.70710678118654746 0.70710678118654757 0]  FollAlignAxisA=+X  BaseAlignAxisA=+Y  FollAlignAxisB=+Y  BaseAlignAxisB=+Z  RotationSequenceAxes=FollowerAxes  RotationSequence=XYX  RotationSequenceAngles=[0 0 0]  RotationSequenceAnglesUnits=deg  RotationMatrix=[1 0 0; 0 1 0; 0 0 1]  Quaternion=[1 0 0 0]
  Transform3 : sm_lib/Frames and Transforms/Rigid Transform  TranslationMethod=Cartesian  TranslationStandardOffset=0  TranslationStandardOffsetUnits=mm  TranslationStandardAxis=+Z  TranslationCartesianOffset=[-181.12877100136708 4.9999999999999627 -105.74999999999996]  TranslationCartesianOffsetUnits=mm  TranslationROffset=0  TranslationROffsetUnits=m  TranslationZOffset=0  TranslationZOffsetUnits=m  TranslationThetaOffset=0  TranslationThetaOffsetUnits=deg  RotationMethod=ArbitraryAxis  RotationAngleUnits=rad  RotationStandardAxis=+Z  RotationAngle=1.7602050674842991  RotationArbitraryAxis=[-0.82650316451596495 -0.3980530863120495 -0.3980530863120495]  FollAlignAxisA=+X  BaseAlignAxisA=+Y  FollAlignAxisB=+Y  BaseAlignAxisB=+Z  RotationSequenceAxes=FollowerAxes  RotationSequence=XYX  RotationSequenceAngles=[0 0 0]  RotationSequenceAnglesUnits=deg  RotationMatrix=[1 0 0; 0 1 0; 0 0 1]  Quaternion=[1 0 0 0]
  Transform4 : sm_lib/Frames and Transforms/Rigid Transform  TranslationMethod=Cartesian  TranslationStandardOffset=0  TranslationStandardOffsetUnits=mm  TranslationStandardAxis=+Z  TranslationCartesianOffset=[-181.12877100136708 4.9999999999999627 -3.2500000000000027]  TranslationCartesianOffsetUnits=mm  TranslationROffset=0  TranslationROffsetUnits=m  TranslationZOffset=0  TranslationZOffsetUnits=m  TranslationThetaOffset=0  TranslationThetaOffsetUnits=deg  RotationMethod=ArbitraryAxis  RotationAngleUnits=rad  RotationStandardAxis=+Z  RotationAngle=1.7602050674842997  RotationArbitraryAxis=[-0.82650316451596506 -0.39805308631204933 -0.39805308631204928]  FollAlignAxisA=+X  BaseAlignAxisA=+Y  FollAlignAxisB=+Y  BaseAlignAxisB=+Z  RotationSequenceAxes=FollowerAxes  RotationSequence=XYX  RotationSequenceAngles=[0 0 0]  RotationSequenceAnglesUnits=deg  RotationMatrix=[1 0 0; 0 1 0; 0 0 1]  Quaternion=[1 0 0 0]
  F : PMIOPort  Side=Left
  F1 : PMIOPort  Port=2  Side=Right
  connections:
  Transform/LConn1 -- ReferenceFrame/RConn1 -- Transform3/LConn1 -- Transform4/LConn1 -- Transform2/LConn1 -- Transform1/LConn1
  Transform/RConn1 -- F/RConn1
  Transform1/RConn1 -- F1/RConn1
  BIELLE_PARALLELOGRAMME_1_RIGID/LConn1 -- Transform2/RConn1
  AXE_BIELLE_1_RIGID/LConn1 -- Transform3/RConn1
  AXE_BIELLE_2_RIGID/LConn1 -- Transform4/RConn1

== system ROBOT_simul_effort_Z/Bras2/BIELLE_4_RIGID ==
  AXE_BIELLE_1_RIGID : Subsystem
  AXE_BIELLE_2_RIGID : Subsystem
  BIELLE_PARALLELOGRAMME_1_RIGID : Subsystem
  ReferenceFrame : sm_lib/Frames and Transforms/Reference Frame
  Transform : sm_lib/Frames and Transforms/Rigid Transform  TranslationMethod=Cartesian  TranslationStandardOffset=0  TranslationStandardOffsetUnits=mm  TranslationStandardAxis=+Z  TranslationCartesianOffset=[-181.12877100136237 13.000000000000043 -105.74999999999874]  TranslationCartesianOffsetUnits=mm  TranslationROffset=0  TranslationROffsetUnits=m  TranslationZOffset=0  TranslationZOffsetUnits=m  TranslationThetaOffset=0  TranslationThetaOffsetUnits=deg  RotationMethod=ArbitraryAxis  RotationAngleUnits=rad  RotationStandardAxis=+Z  RotationAngle=2.0943951023931948  RotationArbitraryAxis=[0.57735026918962562 -0.57735026918962706 0.57735026918962473]  FollAlignAxisA=+X  BaseAlignAxisA=+Y  FollAlignAxisB=+Y  BaseAlignAxisB=+Z  RotationSequenceAxes=FollowerAxes  RotationSequence=XYX  RotationSequenceAngles=[0 0 0]  RotationSequenceAnglesUnits=deg  RotationMatrix=[1 0 0; 0 1 0; 0 0 1]  Quaternion=[1 0 0 0]
  Transform1 : sm_lib/Frames and Transforms/Rigid Transform  TranslationMethod=Cartesian  TranslationStandardOffset=0  TranslationStandardOffsetUnits=mm  TranslationStandardAxis=+Z  TranslationCartesianOffset=[-181.12877100136717 13 -3.2500000000000062]  TranslationCartesianOffsetUnits=mm  TranslationROffset=0  TranslationROffsetUnits=m  TranslationZOffset=0  TranslationZOffsetUnits=m  TranslationThetaOffset=0  TranslationThetaOffsetUnits=deg  RotationMethod=ArbitraryAxis  RotationAngleUnits=rad  RotationStandardAxis=+Z  RotationAngle=2.0943951023931953  RotationArbitraryAxis=[0.57735026918962584 -0.57735026918962562 0.57735026918962595]  FollAlignAxisA=+X  BaseAlignAxisA=+Y  FollAlignAxisB=+Y  BaseAlignAxisB=+Z  RotationSequenceAxes=FollowerAxes  RotationSequence=XYX  RotationSequenceAngles=[0 0 0]  RotationSequenceAnglesUnits=deg  RotationMatrix=[1 0 0; 0 1 0; 0 0 1]  Quaternion=[1 0 0 0]
  Transform2 : sm_lib/Frames and Transforms/Rigid Transform  TranslationMethod=Cartesian  TranslationStandardOffset=0  TranslationStandardOffsetUnits=mm  TranslationStandardAxis=+Z  TranslationCartesianOffset=[-178.12877100136717 5.0000000000000044 -54.5]  TranslationCartesianOffsetUnits=mm  TranslationROffset=0  TranslationROffsetUnits=m  TranslationZOffset=0  TranslationZOffsetUnits=m  TranslationThetaOffset=0  TranslationThetaOffsetUnits=deg  RotationMethod=ArbitraryAxis  RotationAngleUnits=rad  RotationStandardAxis=+Z  RotationAngle=3.1415926535897931  RotationArbitraryAxis=[-0.70710678118654746 0.70710678118654757 -3.9252311467094373e-17]  FollAlignAxisA=+X  BaseAlignAxisA=+Y  FollAlignAxisB=+Y  BaseAlignAxisB=+Z  RotationSequenceAxes=FollowerAxes  RotationSequence=XYX  RotationSequenceAngles=[0 0 0]  RotationSequenceAnglesUnits=deg  RotationMatrix=[1 0 0; 0 1 0; 0 0 1]  Quaternion=[1 0 0 0]
  Transform3 : sm_lib/Frames and Transforms/Rigid Transform  TranslationMethod=Cartesian  TranslationStandardOffset=0  TranslationStandardOffsetUnits=mm  TranslationStandardAxis=+Z  TranslationCartesianOffset=[-181.1287710013672 5.0000000000000044 -105.75000000000003]  TranslationCartesianOffsetUnits=mm  TranslationROffset=0  TranslationROffsetUnits=m  TranslationZOffset=0  TranslationZOffsetUnits=m  TranslationThetaOffset=0  TranslationThetaOffsetUnits=deg  RotationMethod=ArbitraryAxis  RotationAngleUnits=rad  RotationStandardAxis=+Z  RotationAngle=1.7602050674842993  RotationArbitraryAxis=[-0.82650316451596484 -0.39805308631204944 -0.39805308631204939]  FollAlignAxisA=+X  BaseAlignAxisA=+Y  FollAlignAxisB=+Y  BaseAlignAxisB=+Z  RotationSequenceAxes=FollowerAxes  RotationSequence=XYX  RotationSequenceAngles=[0 0 0]  RotationSequenceAnglesUnits=deg  RotationMatrix=[1 0 0; 0 1 0; 0 0 1]  Quaternion=[1 0 0 0]
  Transform4 : sm_lib/Frames and Transforms/Rigid Transform  TranslationMethod=Cartesian  TranslationStandardOffset=0  TranslationStandardOffsetUnits=mm  TranslationStandardAxis=+Z  TranslationCartesianOffset=[-181.12877100136717 5.0000000000000044 -3.2500000000000027]  TranslationCartesianOffsetUnits=mm  TranslationROffset=0  TranslationROffsetUnits=m  TranslationZOffset=0  TranslationZOffsetUnits=m  TranslationThetaOffset=0  TranslationThetaOffsetUnits=deg  RotationMethod=ArbitraryAxis  RotationAngleUnits=rad  RotationStandardAxis=+Z  RotationAngle=1.7602050674842997  RotationArbitraryAxis=[-0.82650316451596506 -0.39805308631204939 -0.39805308631204916]  FollAlignAxisA=+X  BaseAlignAxisA=+Y  FollAlignAxisB=+Y  BaseAlignAxisB=+Z  RotationSequenceAxes=FollowerAxes  RotationSequence=XYX  RotationSequenceAngles=[0 0 0]  RotationSequenceAnglesUnits=deg  RotationMatrix=[1 0 0; 0 1 0; 0 0 1]  Quaternion=[1 0 0 0]
  F : PMIOPort  Side=Left
  F1 : PMIOPort  Port=2  Side=Right
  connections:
  Transform/LConn1 -- ReferenceFrame/RConn1 -- Transform3/LConn1 -- Transform4/LConn1 -- Transform2/LConn1 -- Transform1/LConn1
  Transform/RConn1 -- F/RConn1
  Transform1/RConn1 -- F1/RConn1
  BIELLE_PARALLELOGRAMME_1_RIGID/LConn1 -- Transform2/RConn1
  AXE_BIELLE_1_RIGID/LConn1 -- Transform3/RConn1
  AXE_BIELLE_2_RIGID/LConn1 -- Transform4/RConn1

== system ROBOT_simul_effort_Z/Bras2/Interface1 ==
  Angular Velocity Source : fl_lib/Mechanical/Mechanical Sources/Ideal Angular Velocity Source
  Torque Sensor : fl_lib/Mechanical/Mechanical Sensors/Ideal Torque Sensor
  C : PMIOPort  Side=Left
  T : PMIOPort  Port=2  Side=Right
  w : PMIOPort  Port=3  Side=Right
  R : PMIOPort  Port=4  Side=Left
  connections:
  Angular Velocity Source/RConn1 -- w/RConn1
  C/RConn1 -- Torque Sensor/RConn1
  Torque Sensor/RConn2 -- T/RConn1
  Torque Sensor/LConn1 -- Angular Velocity Source/RConn2
  R/RConn1 -- Angular Velocity Source/LConn1
